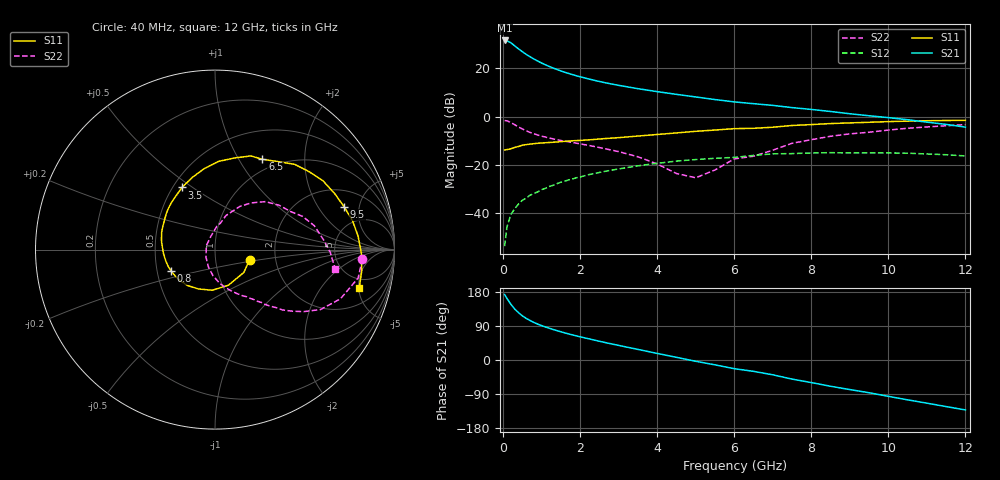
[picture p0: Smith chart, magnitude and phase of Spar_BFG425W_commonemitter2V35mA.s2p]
! Filename: 235bfg425.001
! BFG425W Field C1
! V1=8.753E-001V,V2=2.000E+000V, I1=5.354E-004A, I2=3.494E-002A
# GHz  S  MA  R 50
!  S11  S21  S12  S22
!Freq(GHz)  Mag  Ang  Mag  Ang  Mag  Ang  Mag  Ang
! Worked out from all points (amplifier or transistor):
!   44 points, 40 MHz to 12 GHz, reference 50 ohm
!   highest |S21| = 31.7 dB at 40 MHz (marker M1)
!   |S21| within 3 dB of that: start of sweep to 361.6 MHz
!   unconditionally stable (mu >= 1): start of sweep to 89.16 MHz; 742.6 MHz to end of sweep
!   at 700 MHz: K = 0.98, MSG = 28.8 dB, |S12| = -32.8 dB
!   at 2.4 GHz: K = 1.25, MAG = 16.3 dB, |S12| = -23.6 dB
!   at 12 GHz: K = 1.40, MAG = 2.2 dB, |S12| = -16.4 dB
!   S11 on the Smith chart (normalised r, x): 40 MHz: 1.47, -0.17; 800 MHz: 0.59, -0.15; 3.5 GHz: 0.56, +0.45; 6.5 GHz: 0.85, +1.27; 9.5 GHz: 3.14, +3.52; 12 GHz: 3.59, -5.06
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0.04  0.201 -16.5  38.26 172.6  0.002 72.0  0.823 -3.6
0.1  0.205 -38.4  37.57 162.7  0.005 79.2  0.813 -11.2
0.2  0.212 -69.4  34.45 147.2  0.009 72.5  0.751 -21.4
0.3  0.227 -93.9  29.61 134.7  0.012 69.6  0.676 -29.6
0.4  0.238 -112.9  25.63 124.9  0.015 66.8  0.604 -34.9
0.5  0.252 -127.5  22.34 116.5  0.018 64.9  0.55 -38.6
0.6  0.26 -138.2  19.66 109.9  0.02 64.1  0.504 -41.8
0.7  0.266 -146.5  17.54 104.3  0.023 63.3  0.466 -43.8
0.8  0.272 -154.0  15.74 99.1  0.025 62.9  0.439 -45.8
1  0.281 -166.1  12.97 90.8  0.03 61.6  0.39 -48.8
1.3  0.291 179.9  10.2 80.5  0.037 59.4  0.343 -53.2
1.7  0.307 165.7  7.885 68.8  0.048 55.9  0.297 -59.6
2.2  0.325 150.4  6.109 56.6  0.061 50.1  0.252 -67.6
2.8  0.354 134.5  4.776 42.8  0.076 42.2  0.201 -78.9
3.5  0.392 118.0  3.794 27.9  0.094 32.1  0.145 -94.7
4.5  0.455 97.6  2.891 7.0  0.118 16.6  0.065 -141.0
5.5  0.522 77.9  2.253 -12.8  0.135 0.7  0.077 107.7
6.5  0.568 62.3  1.848 -29.9  0.155 -12.2  0.149 78.8
8.5  0.713 32.7  1.272 -69.3  0.177 -48.4  0.388 43.5
9.5  0.758 18.3  1.036 -86.3  0.174 -64.5  0.47 26.9
10.5  0.801 5.3  0.857 -105.2  0.172 -82.4  0.569 13.5
12  0.832 -15.1  0.6 -131.8  0.151 -111.0  0.678 -9.0
